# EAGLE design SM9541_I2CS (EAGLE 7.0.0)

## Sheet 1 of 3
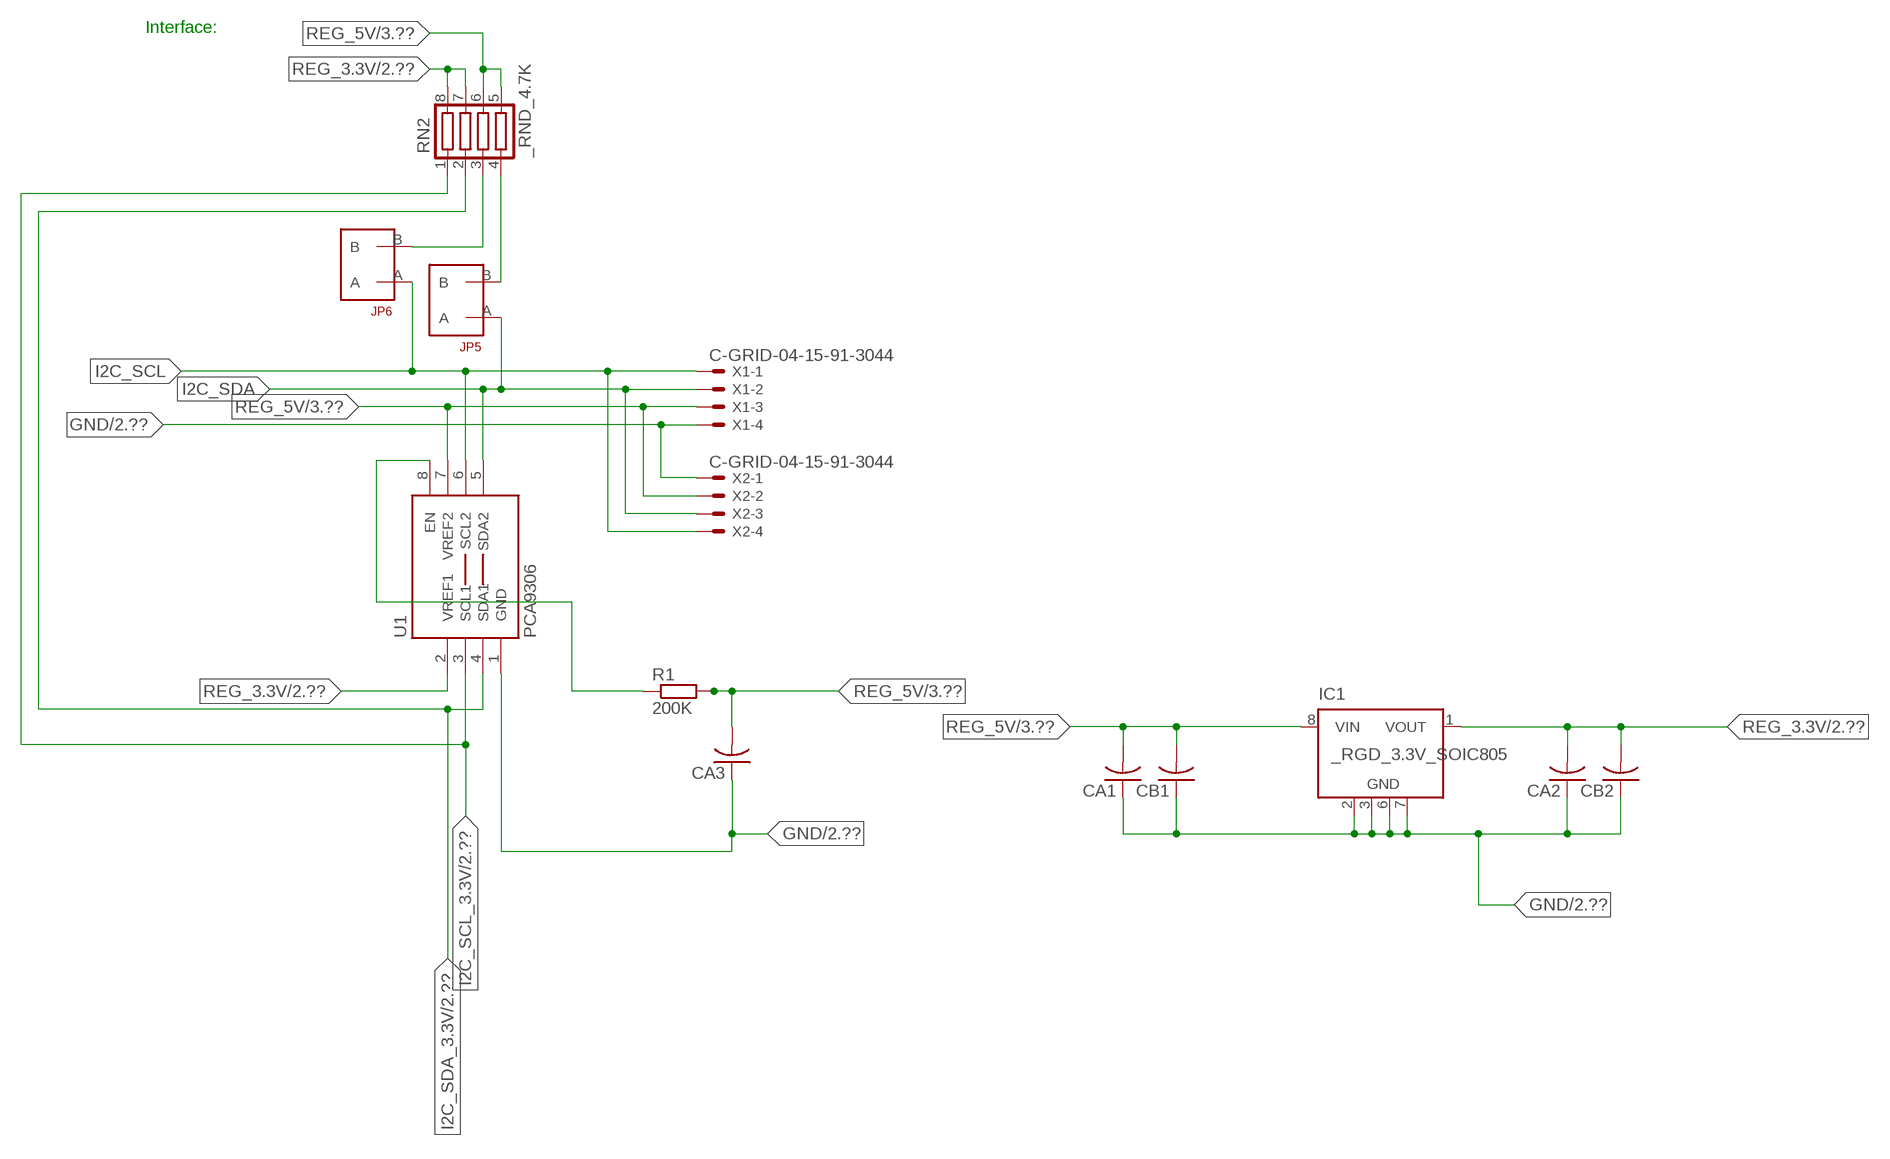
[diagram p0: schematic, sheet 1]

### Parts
CA1  CC1206KRX7R9BB104  [.1UF]
CA2  CC1206KRX7R9BB104  [.1UF]
CA3  CC1206KRX7R9BB104  [.1UF]
CB1  TMK316F106ZL-TC1206K  [TMK316F106ZL-T]
CB2  TMK316F106ZL-TC1206K  [TMK316F106ZL-T]
IC1  _RGD_3.3V_SOIC805  [_RGC_3.3V_SOIC8]
JP5  JUMPER_1X2_2MM  [JUMPER_1X2_2MM]
JP6  JUMPER_1X2_2MM  [JUMPER_1X2_2MM]
R1  200K  RESISTOR_SMT-0603  [R603]
RN2  _RND_4.7K  [RND]
U1  PCA9306  PCA9306_NCD  [PSOP-8]
X1  C-GRID-04-15-91-3044  [15-91-04]
X2  C-GRID-04-15-91-3044  [15-91-04]

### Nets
GND: CA1.1 CA2.1 CA3.1 CB1.1 CB2.1 IC1.2(GND) IC1.3(GND) IC1.6(GND) IC1.7(GND) U1.1(GND) X1.4 X2.1 ; also sheet 2,3
I2C_SCL: JP6.A U1.6(SCL2) X1.1 X2.4
I2C_SCL_3.3V: RN2.1 U1.3(SCL1) ; also sheet 2
I2C_SDA: JP5.A U1.5(SDA2) X1.2 X2.3
I2C_SDA_3.3V: RN2.2 U1.4(SDA1) ; also sheet 2
N$1: JP6.B RN2.3
N$2: JP5.B RN2.4
N$23: R1.1 U1.8(EN)
REG_3.3V: CA2.2 CB2.2 IC1.1(VOUT) RN2.7 RN2.8 U1.2(VREF1) ; also sheet 2
REG_5V: CA1.2 CA3.2 CB1.2 IC1.8(VIN) R1.2 RN2.5 RN2.6 U1.7(VREF2) X1.3 X2.2 ; also sheet 3
Unconnected: IC1.4(NC) IC1.5(NC)

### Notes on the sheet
- Interface:

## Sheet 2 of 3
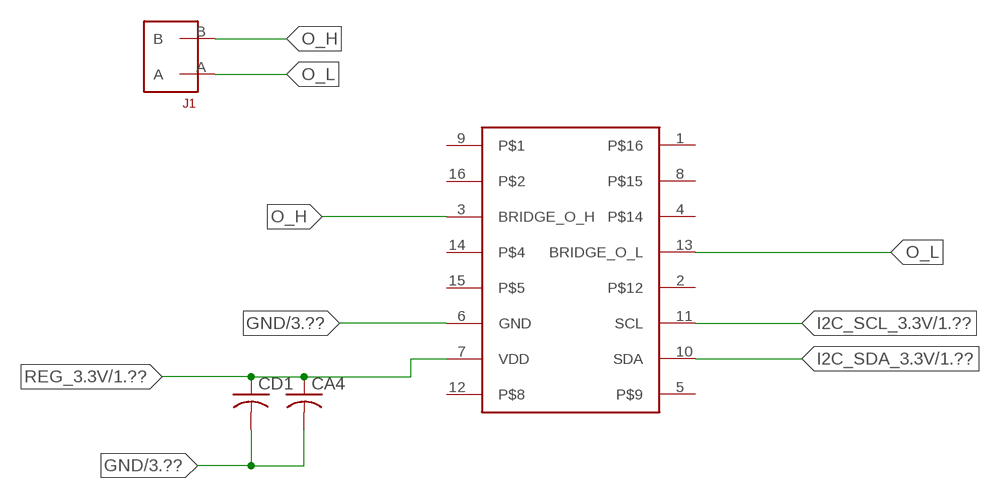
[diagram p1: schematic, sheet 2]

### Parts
CA4  _CA_.10UF_50VC1206K  [_CA_.1UF_50V]
CD1  _CD_10NF_50VC1206K  [_CD_10NF_50V]
J1  JUMPER_1X2_2MM  [JUMPER_1X2_2MM]
U2  SM9541  [16-SOIC]

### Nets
GND: CA4.2 CD1.2 U2.6(GND) ; also sheet 1,3
I2C_SCL_3.3V: U2.11(SCL) ; also sheet 1
I2C_SDA_3.3V: U2.10(SDA) ; also sheet 1
O_H: J1.B U2.3(BRIDGE_O_H)
O_L: J1.A U2.13(BRIDGE_O_L)
REG_3.3V: CA4.1 CD1.1 U2.7(VDD) ; also sheet 1
Unconnected: U2.1 U2.2 U2.4 U2.5 U2.8 U2.9 U2.12 U2.14 U2.15 U2.16

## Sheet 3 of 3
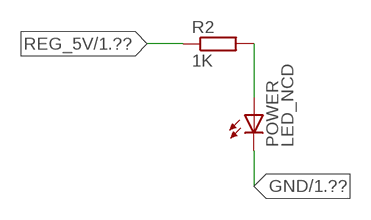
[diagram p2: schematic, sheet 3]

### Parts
POWER  LED_NCD  [CHIPLED_0603]
R2  1K  RESISTOR_SMT-0402  [R402]

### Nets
GND: POWER.C ; also sheet 1,2
N$4: POWER.A R2.2
REG_5V: R2.1 ; also sheet 1

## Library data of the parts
CA1-CA3 = NCD_ULTIMATE_LIBRARY:CC1206KRX7R9BB104: Capacitor CA .1uF 50V SMT C1206K CC1206KRX7R9BB104
CA4 = NCD_ULTIMATE_LIBRARY:_CA_.10UF_50V: Capacitor .1uF SMT
CB1 CB2 = NCD_ULTIMATE_LIBRARY:TMK316F106ZL-T: Capacitor CB 10uF SMT 1206 TMK316F106ZL-T
CD1 = NCD_ULTIMATE_LIBRARY:_CD_10NF_50V: Capacitor 10nF SMT
IC1 = NCD_ULTIMATE_LIBRARY:_RGD_3.3V_SOIC8: Regulator Linear 3.3V Chip Positive VOLTAGE REGULATOR Digikey 497-1199-2-ND/L78L33ACD13TR
J1 JP5 JP6 = NCD_ULTIMATE_CONNECTORS:JUMPER_1X2_2MM
POWER = NCD_ULTIMATE_LIBRARY:LED_NCD: LED Digikey 754-1132-2-ND/APT2012SRCPRV
R1 R2 = NCD_ULTIMATE_LIBRARY:RESISTOR_SMT: NCD Resistor
RN2 = NCD_ULTIMATE_LIBRARY:_RND_4.7K: Resistor Array RND SMT 4.7K x 4 Single Resistor Source: http://www.ctscorp.com/components/Datasheets/CTSChipArrayDs.pdf Digikey 742C083472JPTR-ND/742C083472JP; OC_FARNELL: unknown; OC_NEWARK: unknown
U1 = NCD_ULTIMATE_LIBRARY:PCA9306_NCD: NCD Bidirectional I2C level shifter. NOT compatible with all available part number pinout schemes- DOUBLE CHECK!!!; PROD_ID: IC-10023
U2 = NCD_ULTIMATE_bhaskar:SM9541
X1 X2 = NCD_ULTIMATE_CONNECTORS:C-GRID-04: CONNECTOR 4-Pos I2C wire to board 2.54 mm (0.100") pitch header Digikey WM1342-ND/0015912045; OC_FARNELL: unknown; OC_NEWARK: unknown

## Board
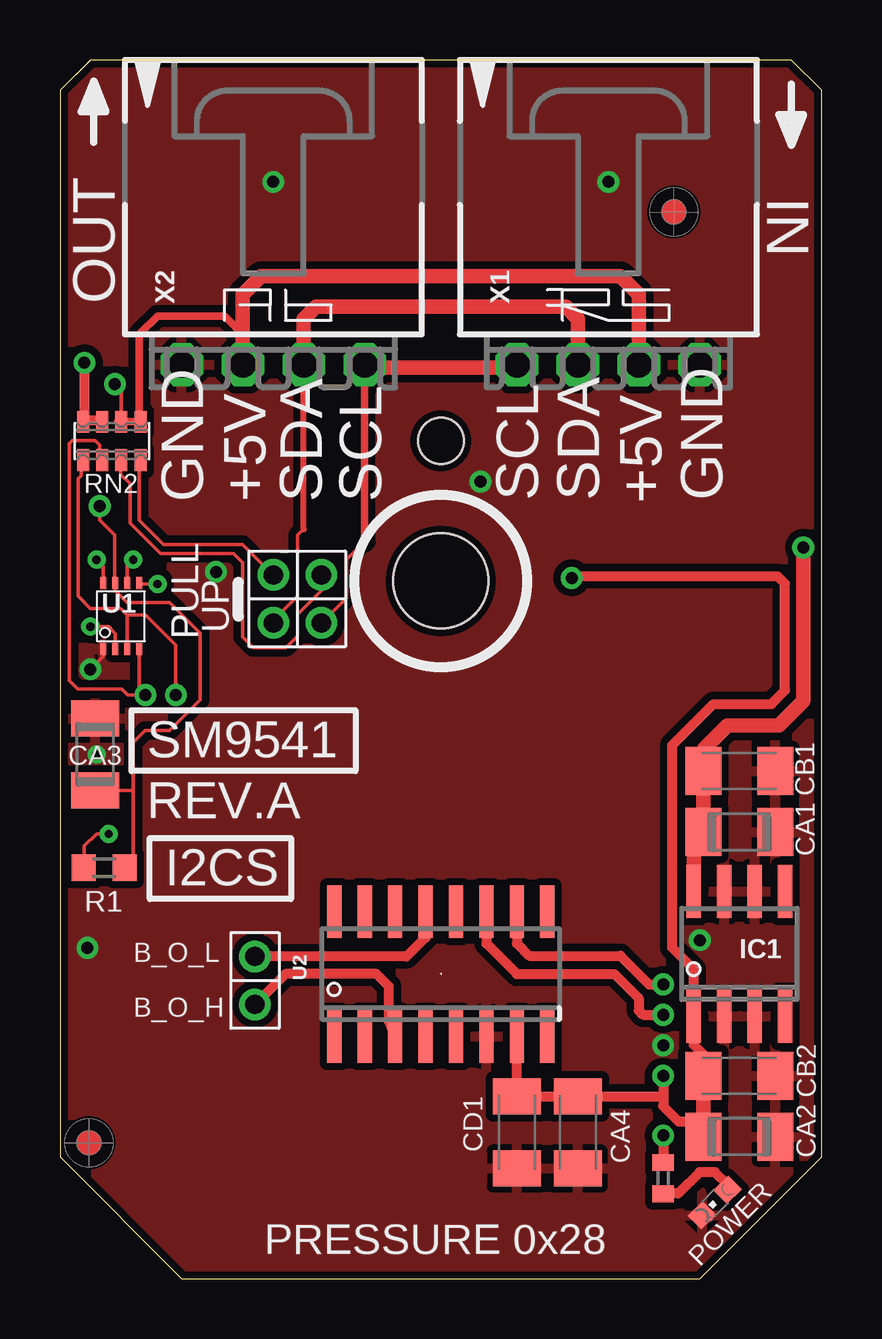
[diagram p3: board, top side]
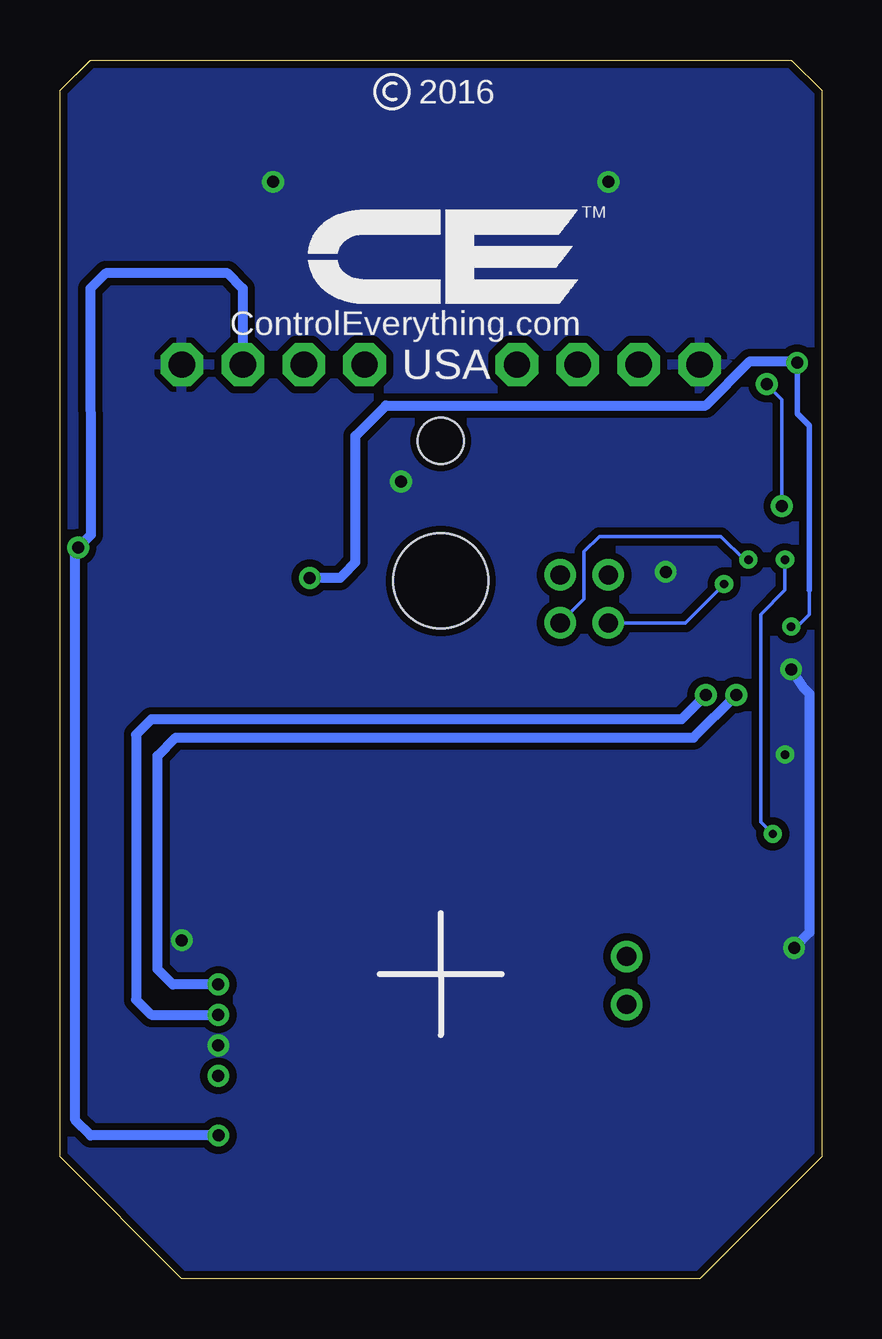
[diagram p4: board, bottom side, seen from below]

Size 31.75 x 50.8 mm. Coordinates in mm from the lower left corner, seen from the top.
Outline: 48 segments
Copper layers (1*16): Top 0.035mm / dielectric 1.5mm / Bottom 0.035mm
Design rules "default": minimum track width 5mil, minimum drill 24mil, track to track 5mil, track to pad 5mil, pad to pad 5mil, via to via 5mil, smd to smd 5mil, copper to edge 10mil, drill to drill 8mil, minimum pad ring 10mil, minimum via ring 8mil, stop-mask expansion 2mil, vias tented up to drill 0mil, thermal gap 10mil
Holes 3.96 mm at 15.88,29.08
Holes 1.91 mm at 15.88,34.93

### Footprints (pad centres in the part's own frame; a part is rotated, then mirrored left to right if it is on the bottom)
.1UF = smd 1.5 x 2: 1 -1.5,0; 2 1.5,0
_CA_.1UF_50V = smd 1.5 x 2: 1 -1.5,0; 2 1.5,0
TMK316F106ZL-T = smd 1.5 x 2: 1 -1.5,0; 2 1.5,0
_CD_10NF_50V = smd 1.5 x 2: 1 -1.5,0; 2 1.5,0
_RGC_3.3V_SOIC8 = smd 0.6 x 2.2: 1 -1.905,-2.6; 2 -0.635,-2.6; 3 0.635,-2.6; 4 1.905,-2.6; 5 1.905,2.6; 6 0.635,2.6; 7 -0.635,2.6; 8 -1.905,2.6
JUMPER_1X2_2MM = drill 0.8: A 0,2; B 0,0
CHIPLED_0603 = smd 0.8 x 0.876: A 0,-0.75; C 0,0.75
R603 = smd 1 x 1.1: 1 -0.85,0; 2 0.85,0
R402 = smd 0.7 x 0.9: 1 -0.65,0; 2 0.65,0
RND = smd 0.5 x 0.9: 1 -1.2,-0.8; 2 -0.4,-0.8; 3 0.4,-0.8; 4 1.2,-0.8; 5 1.2,0.8; 6 0.4,0.8; 7 -0.4,0.8; 8 -1.2,0.8
PSOP-8 = smd 0.25 x 0.5: 1 -0.73,-1.37; 2 -0.23,-1.37; 3 0.27,-1.37; 4 0.77,-1.37; 5 0.77,1.38; 6 0.27,1.38; 7 -0.23,1.38; 8 -0.73,1.38
16-SOIC = smd 0.6 x 2.2: 1 -4.445,-2.6; 2 -3.175,-2.6; 3 -1.905,-2.6; 4 -0.635,-2.6; 5 0.635,-2.6; 6 1.905,-2.6; 7 3.175,-2.6; 8 4.445,-2.6; 9 4.445,2.6; 10 3.175,2.6; 11 1.905,2.6; 12 0.635,2.6; 13 -0.635,2.6; 14 -1.905,2.6; 15 -3.175,2.6; 16 -4.445,2.6
15-91-04 = drill 1.1 pad 1.778 octagon: 1 -3.81,-7.62; 2 -1.27,-7.62; 3 1.27,-7.62; 4 3.81,-7.62

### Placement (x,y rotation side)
CA1  28.32,18.62 180 top
CA2  28.32,5.92 180 top
CA3  1.46,21.86 270 top
CA4  21.59,6.1 270 top
CB1  28.32,21.16 180 top
CB2  28.32,8.46 180 top
CD1  19.05,6.1 270 top
IC1  28.32,13.54 0 top
J1  8.13,11.43 0 top
JP5  8.89,29.34 180 top
JP6  10.9,29.34 180 top
POWER  27.3,3.18 135 top
R1  1.84,17.13 0 top
R2  25.15,4.19 270 top
RN2  2.16,34.93 0 top
U1  2.54,27.61 0 top
U2  15.88,12.7 0 top
U$5  [VISION_REF10]  1.21,5.66 90 top
U$28  [VISION_REF10]  25.59,44.46 90 top
X1  22.86,45.72 0 top
X2  8.89,45.72 0 top

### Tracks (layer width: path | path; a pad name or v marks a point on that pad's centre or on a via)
GND  (via drill 0.35, 0.5)
  Top 0.152: CA3.1 1.52,23.42 1.52,23.62 | v1.27,25.4 1.81,25.94 U1.1
  Bottom 0.406: v1.27,25.4 0.76,24.64 0.51,24.38 0.51,14.43 v1.15,13.79
  other vias: 8.89,45.72 22.86,45.72 25.15,9.73 17.53,33.22 26.67,14.11 6.5,29.46 1.52,21.84
  pour Bottom (isolate 0.305): -0.64,5.08 -0.64,49.53 1.27,51.44 30.48,51.44 32.38,49.53 32.38,5.08 26.67,-0.63 5.08,-0.63
  pour Top (isolate 0.305): 4.45,-1.27 -1.27,4.45 -1.27,50.17 0.64,52.07 31.11,52.07 33.02,50.17 33.02,4.45 27.3,-1.27
I2C_SCL  (via drill 0.35)
  Top 0.152: 12.7,30.73 11.94,29.97 11.94,28.38 JP6.A | v3.05,29.97 2.81,29.73 U1.6
  Top 0.305: 12.7,30.73 X2.4
  Top 0.406: X2.4 12.7,37.97 | 19.05,37.97 X1.1
  Top 0.61: 12.7,37.97 19.05,37.97
  Bottom 0.152: JP6.A 9.91,28.33 9.91,30.3 9.27,30.94 4.19,30.94 3.23,29.97 v3.05,29.97
I2C_SCL_3.3V  (via drill 0.5)
  Top 0.152: RN2.1 0.89,34.07 0.89,33.48 0.77,33.35 0.77,29.1 0.76,29.09 0.76,28.45 1.27,27.94 2.54,27.94 2.81,27.67 | 2.81,27.67 U1.3 | v4.83,24.33 v4.83,24.34 4.83,26.42 3.57,27.67 2.81,27.67
  Top 0.406: 17.78,15.68 U2.11 17.78,13.97 19.05,12.7 23.11,12.7 24.13,11.68 24.13,11.18 24.31,11 v25.15,11
  Bottom 0.406: v4.83,24.33 5.84,23.32 27.94,23.32 28.58,22.68 28.58,11.63 27.94,11 v25.15,11
I2C_SDA  (via drill 0.35)
  Top 0.152: JP5.A 8.89,27.44 9.91,28.45 9.91,30.99 10.16,31.24 | U1.5 3.34,28.96 v4.06,28.96
  Top 0.254: 10.16,31.24 10.16,31.25 X2.3
  Top 0.61: X2.3 10.16,40.01 10.67,40.51 21.09,40.51 21.59,40.01 X1.2
  Bottom 0.152: v4.06,28.96 5.68,27.34 JP5.A
I2C_SDA_3.3V  (via drill 0.5)
  Top 0.152: RN2.2 1.65,34.14 1.65,34.75 1.46,34.94 0.51,34.94 0.38,34.81 0.38,26.37 0.38,26.36 0.38,24.94 0.74,24.59 2.56,24.59 2.82,24.33 v3.56,24.33 3.31,24.58 U1.4
  Top 0.406: 19.05,15.81 U2.10 19.05,13.97 19.56,13.46 23.37,13.46 24.56,12.27 v25.15,12.27
  Bottom 0.406: v25.15,12.27 27.05,12.27 27.69,12.9 27.69,21.79 26.93,22.56 5.34,22.56 v3.56,24.33
N$1
  Top 0.152: JP6.B 10.92,29.31 10.92,28.7 9.91,27.69 9.91,26.8 9.42,26.31 8.06,26.31 7.62,26.75 7.62,29.84 7.24,30.23 4.19,30.23 2.92,31.5 2.92,33.15 2.54,33.53 2.54,34.1 RN2.3
  Top 0.305: 2.54,34.02 RN2.3
N$2
  Top 0.152: JP5.B 7.62,30.61 4.32,30.61 3.3,31.62 3.3,34.07 RN2.4
  Top 0.305: 3.37,33.88 RN2.4
N$4
  Top 0.406: POWER.A 27.84,3.92 27.3,4.45 26.67,4.45 25.78,3.56 25.16,3.56 R2.2
N$23  (via drill 0.35)
  Top 0.152: R1.1 1.02,17.16 1.02,18.03 1.52,18.54 v2.03,18.54 | v1.52,29.97 1.81,29.69 U1.8
  Bottom 0.152: v2.03,18.54 2.54,19.05 2.54,27.69 1.52,28.7 v1.52,29.97
O_H
  Top 0.406: U2.3 13.72,10.74 13.72,12.19 13.21,12.7 9.4,12.7 J1.B
O_L
  Top 0.406: 15.24,15.68 U2.13 15.24,14.22 14.45,13.43 J1.A
REG_3.3V  (via drill 0.35, 0.5)
  Top 0.152: v1.27,27.18 2.03,27.18 2.31,26.9 U1.2
  Top 0.406: CB2.2 26.82,9.35 26.42,9.75 26.42,10.36 | v25.15,8.46 25.15,7.6 | 25.15,7.6 25.15,7.19 25.78,6.55 26.82,6.55 | IC1.1 26.42,12.9 25.53,13.79 25.53,22.24 27.24,23.95 29.66,23.95 30.23,24.52 30.23,28.97 29.91,29.29 21.41,29.29 v21.34,29.21 | 26.52,5.62 CA2.2 | v1.02,38.18 1.02,35.78 | 1.02,35.78 RN2.8 | 1.02,35.78 1.71,35.78 RN2.7 | 25.15,7.6 CA4.1 CD1.1 U2.7
  Top 0.61: CB2.2 26.82,6.55 CA2.2 | 26.42,10.36 IC1.1
  Bottom 0.152: 0.51,28.7 0.51,27.69 1.02,27.18 v1.27,27.18
  Bottom 0.229: 0.51,28.7 0.51,35.56 1.02,36.07 v1.02,38.18
  Bottom 0.406: v1.02,38.18 1.08,38.24 2.99,38.24 4.83,36.4 18.16,36.4 19.43,35.13 19.43,29.87 19.94,29.34 20.07,29.21 v21.34,29.21
REG_5V  (via drill 0.5)
  Top 0.152: RN2.6 2.56,37.01 v2.29,37.29 | R1.2 3.05,17.49 3.05,20.36 | 3.05,20.36 3.05,22.35 3.56,22.86 4.57,22.86 5.84,24.13 5.84,26.92 4.57,28.19 2.79,28.19 2.31,28.68 U1.7 2.29,29.01 2.29,30.99 1.65,31.62 v1.65,32.21 | CA3.2 3.05,20.36
  Top 0.305: 7.62,39.37 7.5,39.37 | 2.42,35.74 RN2.6 RN2.5 3.31,35.8 3.31,39.37 4.07,40.13 6.86,40.13 7.62,39.37 | X2.2 7.62,39.37
  Top 0.406: v25.15,5.97 R2.1 | 24.13,41.02 X1.3
  Top 0.61: X2.2 7.62,41.02 8.38,41.78 23.37,41.78 24.13,41.02 24.13,38.23 | IC1.8 26.42,18.21 CA1.2 CB1.2 26.86,21.2 26.86,22.11 27.82,23.06 29.98,23.06 30.99,24.08 v30.99,30.48
  Bottom 0.152: v1.65,32.21 1.65,36.65 v2.29,37.29
  Bottom 0.406: v25.15,5.97 30.48,5.97 31.11,6.6 31.11,30.36 v30.99,30.48 30.47,31 30.48,41.27 29.84,41.91 24.77,41.91 24.13,41.28 X1.3

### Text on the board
tNames: IN | OUT | GND | +5V | SDA | SCL | SCL | SDA | +5V | GND | PULL | UP | SM9541 | REV.A | I2CS | B_O_L | B_O_H | PRESSURE 0x28
bNames: 2016 | TM | ControlEverything.com | USA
